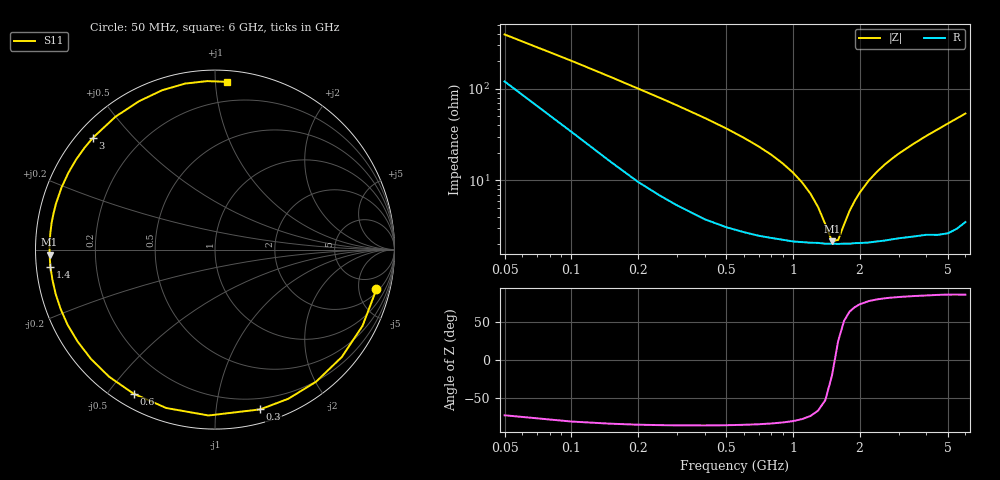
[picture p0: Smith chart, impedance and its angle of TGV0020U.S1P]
! SIEMENS Discrete & RF Semiconductors
! BAT64
! Si Schottky Diode in SOT23
! IF = 0.02 mA
! S-Parameters:  February  1997
# GHz  S  MA  R  50
!  f  S11
! GHz  MAG  ANG
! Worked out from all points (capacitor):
!   34 points, 50 MHz to 6 GHz, reference 50 ohm
!   read as one part to ground: C = 7.91 pF near 50 MHz
!   lowest |Z| = 2.16 ohm at 1.5 GHz (marker M1)
!   series resonance near 1.544 GHz, so ESL is about 1.3 nH
!   S11 on the Smith chart (normalised r, x): 50 MHz: 2.41, -7.50; 300 MHz: 0.11, -1.32; 600 MHz: 0.05, -0.58; 1.4 GHz: 0.04, -0.05; 3 GHz: 0.05, +0.39; 6 GHz: 0.07, +1.07
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0.05  0.9262 -13.8
0.1  0.9252 -27.3
0.15  0.9258 -40.3
0.2  0.9268 -52.6
0.25  0.926 -63.8
0.3  0.9252 -74.2
0.4  0.9249 -92.2
0.5  0.9234 -107.1
0.6  0.9221 -119.5
0.7  0.9218 -129.8
0.8  0.9212 -138.6
0.9  0.9211 -146.3
1  0.922 -153.0
1.1  0.9216 -159.0
1.2  0.9216 -164.4
1.4  0.9223 -174.0
1.5  0.922 -178.3
1.6  0.9225 177.8
2  0.9222 164.0
2.4  0.9222 152.3
2.6  0.9223 147.0
3  0.9224 137.4
3.5  0.9251 126.8
4  0.9287 117.1
4.5  0.9355 108.4
5  0.9398 100.2
5.5  0.9398 92.7
6  0.9372 85.8
